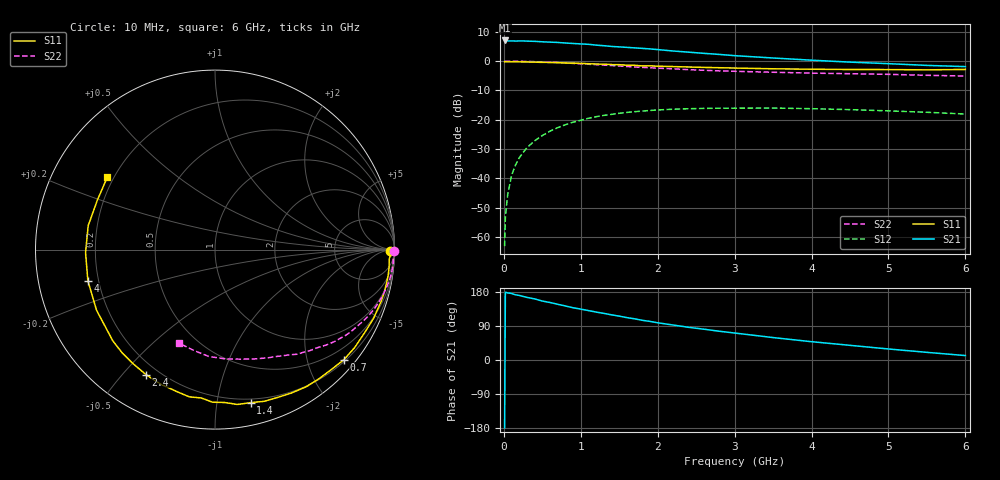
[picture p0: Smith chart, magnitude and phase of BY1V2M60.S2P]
! SIEMENS Small Signal Semiconductors
! BFY420
! Si NPN RF SIEGET Grounded Emitter Transistor in MICRO-X
! VCE = 1.25 V  IC = 0.6 mA
! Common Emitter S-Parameters:  October  1996
# GHz  S  MA  R  50
!  f  S11  S21  S12  S22
! GHz  MAG  ANG  MAG  ANG  MAG  ANG  MAG  ANG
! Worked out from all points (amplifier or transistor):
!   36 points, 10 MHz to 6 GHz, reference 50 ohm
!   highest |S21| = 7.1 dB at 10 MHz (marker M1)
!   |S21| within 3 dB of that: start of sweep to 1.952 GHz
!   unconditionally stable (mu >= 1): 4.7 GHz to end of sweep
!   at 250 MHz: K = 0.04, MSG = 19.0 dB, |S12| = -31.2 dB
!   at 1.4 GHz: K = 0.21, MSG = 11.6 dB, |S12| = -18.1 dB
!   at 6 GHz: K = 1.37, MAG = 4.5 dB, |S12| = -18.0 dB
!   S11 on the Smith chart (normalised r, x): 10 MHz: 72, -33; 700 MHz: 0.24, -2.69; 1.4 GHz: 0.17, -1.25; 2.4 GHz: 0.15, -0.58; 4 GHz: 0.16, -0.12; 6 GHz: 0.18, +0.30
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0.01  0.9774 -0.6  2.256 -179.2  0.0007 95.4  0.9989 -0.3
0.02  0.9802 -1.4  2.255 178.7  0.0022 79.4  0.9999 -0.6
0.05  0.9723 -3.0  2.215 177.1  0.0053 89.9  0.998 -1.5
0.1  0.9752 -6.0  2.218 175.6  0.0112 87.2  0.9947 -3.1
0.15  0.9754 -8.8  2.204 172.1  0.0168 83.7  0.9952 -4.6
0.2  0.9734 -11.8  2.212 170.5  0.0225 83.7  0.9946 -6.0
0.25  0.9723 -14.6  2.215 167.8  0.0276 80.2  0.9916 -7.5
0.4  0.963 -23.5  2.179 161.3  0.0438 74.6  0.9806 -12.0
0.5  0.9533 -29.3  2.141 155.6  0.0539 71.4  0.9701 -14.9
0.7  0.9444 -40.5  2.086 147.1  0.0735 64.1  0.9463 -20.5
0.9  0.9235 -51.4  2.003 137.9  0.0912 57.0  0.9171 -25.7
1.1  0.9051 -62.1  1.939 130.4  0.1063 50.4  0.8869 -30.7
1.4  0.8755 -76.9  1.783 119.2  0.1238 41.2  0.843 -37.2
1.8  0.83 -95.3  1.653 104.7  0.1408 30.6  0.784 -44.7
2.2  0.8092 -111.7  1.491 92.3  0.1516 21.2  0.7416 -51.8
2.4  0.7956 -118.9  1.425 86.3  0.1545 17.5  0.7163 -55.0
2.8  0.7736 -132.0  1.304 75.9  0.1579 10.3  0.6826 -60.9
3.5  0.7415 -152.9  1.133 59.2  0.1589 0.2  0.6473 -70.3
4  0.7292 -166.3  1.04 48.3  0.1547 -5.7  0.6254 -77.4
4.5  0.7214 -178.6  0.963 38.7  0.1492 -11.0  0.6113 -84.8
5.5  0.711 157.2  0.847 20.2  0.1344 -17.6  0.5742 -101.8
6  0.7232 146.0  0.808 11.7  0.1254 -18.6  0.558 -111.3
